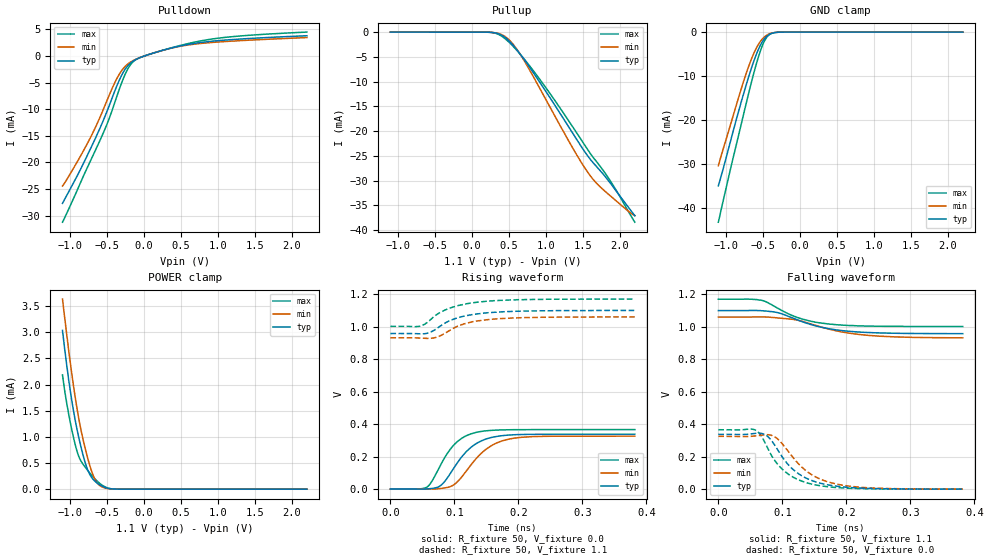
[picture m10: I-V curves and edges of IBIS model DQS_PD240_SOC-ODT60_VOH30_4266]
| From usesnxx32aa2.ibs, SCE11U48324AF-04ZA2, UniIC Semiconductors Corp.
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| DQS_PD240_SOC-ODT60_VOH30_4266
| (240 Ohm Pulldown, 60 Ohm System ODT Setting, VOH=VDDQ/3.0, 3200-4266Mbps)
[Model]   DQS_PD240_SOC-ODT60_VOH30_4266
Model_type   I/O
Vinl = 123.333mV
Vinh = 243.333mV
Vmeas = 183.333mV
Vref = 0.0mV
Cref = 0.0pF
Rref = 60.000Ohm
|   typ   min   max
|C_comp   0.838pF   0.788pF   0.888pF
C_comp_pullup   0.4190pF   0.3940pF   0.4440pF
C_comp_pulldown   0.4190pF   0.3940pF   0.4440pF
| Note: C_comp changes when the ODT circuit is enabled.
[Model Spec]
| Input threshold voltage corners
Vinl   0.1233V   0.1167V   0.1350V
Vinh   0.2433V   0.2367V   0.2550V
| Measurement voltage corners
Vmeas   0.1833V   0.1767V   0.1950V
| Timing spec test load voltage corners
Vref   0.0000V   0.0000V   0.0000V
| Dynamic Overshoot Parameters from LPDDR4 Specification
D_overshoot_ampl_h   0.30   NA   NA
D_overshoot_ampl_l   0.30   NA   NA
D_overshoot_area_h   0.1n   NA   NA
D_overshoot_area_l   0.1n   NA   NA
[Receiver Thresholds]
Vcross_low   = 123.3mV
Vcross_high  = 243.3mV
Vdiff_ac   = 120mV
Vdiff_dc   = 120mV
Tdiffslew_ac = 10.000ns |Not specified, so set to high value
[Voltage Range]   1.1000V   1.0600V   1.1700V
[Pullup Reference]   1.1000V   1.0600V   1.1700V
| Junction Temperature (Ambient temp is 35C typ 95C min -40C max)
[Temperature Range]   50.0   110.0   -40.0
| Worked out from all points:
|   slope of the pulldown table from 0 to 0.165 V, typ, clamps not added: 223 ohm
|   slope of the pullup table from 0 to 0.165 V, typ, clamps not added: 19.4 kohm
|   GND clamp passes 1 mA (typ) near -0.45 V on its own axis
|   POWER clamp passes 1 mA (typ) near -0.88 V on its own axis
|   rising waveform, R_fixture 50, V_fixture 0.0: 20-80 % time 41.5ps typ, 45.6ps min, 36.3ps max; typ from 0.001 V to 0.338 V
|   falling waveform, R_fixture 50, V_fixture 1.1: 20-80 % time 70.4ps typ, 79.9ps min, 60.1ps max; typ from 1.1 V to 0.958 V
|   rising waveform, R_fixture 50, V_fixture 1.1: 20-80 % time 51.9ps typ, 50ps min, 52.9ps max; typ from 0.958 V to 1.1 V
|   falling waveform, R_fixture 50, V_fixture 0.0: 20-80 % time 49.1ps typ, 53.6ps min, 45.1ps max; typ from 0.338 V to 0.001 V
[Pulldown]
|   Voltage   I(typ)   I(min)   I(max)
-1.1V     -27.71mA   -24.44mA   -31.25mA
-918.5mV  -22.98mA   -20.31mA   -25.78mA
-720.5mV  -17.39mA   -15.27mA   -19.65mA
-499.4mV  -10.41mA   -8.375mA   -12.82mA
-347.6mV  -5.002mA   -3.762mA   -6.827mA
-232.1mV  -2.055mA   -1.662mA   -2.791mA
-129.8mV  -798.7uA   -738.7uA   -879.6uA
0V        -19.07uA   -16.89uA   -13.69uA
394.9mV   1.594mA    1.561mA    1.646mA
843.7mV   2.68mA     2.468mA    3.039mA
1.395V    3.278mA    2.967mA    3.877mA
2.2V      3.818mA    3.475mA    4.505mA
[GND Clamp]
|   Voltage   I(typ)   I(min)   I(max)
-1.1V     -34.88mA   -30.34mA   -43.13mA
-944.9mV  -25.34mA   -21.53mA   -31.71mA
-789.8mV  -15.79mA   -12.83mA   -20.82mA
-723.8mV  -11.98mA   -9.381mA   -16.18mA
-664.4mV  -8.768mA   -6.598mA   -12.12mA
-588.5mV  -5.128mA   -3.689mA   -7.33mA
-522.5mV  -2.67mA    -1.906mA   -3.822mA
-466.4mV  -1.297mA   -942.8uA   -1.695mA
-413.6mV  -567.5uA   -419uA     -621.4uA
-354.2mV  -179.7uA   -135.9uA   -159.4uA
-258.5mV  -16.1uA    -14.2uA    -9.795uA
2.2V      0A         0A         0A
[Pullup]
|   Voltage   I(typ)   I(min)   I(max)
-1.1V     4.189uA    6.456uA    1.888uA
229.9mV   -30.52uA   -30.79uA   -31.1uA
332.2mV   -215.1uA   -179.7uA   -295.5uA
437.8mV   -961.7uA   -787.6uA   -1.21mA
553.3mV   -2.603mA   -2.4mA     -2.822mA
691.9mV   -5.249mA   -5.417mA   -5.187mA
1.075V    -13.73mA   -15.72mA   -12.85mA
1.411V    -21.61mA   -24.71mA   -20.28mA
1.576V    -25.28mA   -28.59mA   -24.04mA
1.695V    -27.39mA   -30.74mA   -26.42mA
1.89V     -30.93mA   -33.36mA   -30.56mA
2.2V      -37.14mA   -37.08mA   -38.43mA
[POWER Clamp]
|   Voltage   I(typ)   I(min)   I(max)
-1.1V     3.036mA    3.636mA    2.186mA
-1.041V   2.347mA    2.931mA    1.626mA
-981.2mV  1.754mA    2.277mA    1.183mA
-918.5mV  1.248mA    1.669mA    798.4uA
-859.1mV  857.6uA    1.195mA    561uA
-793.1mV  506.3uA    776.1uA    421uA
-740.3mV  306.1uA    494.5uA    324.3uA
-667.7mV  159.9uA    206.2uA    205.2uA
-598.4mV  83.67uA    71.98uA    113.1uA
-502.7mV  22.64uA    13.95uA    29.28uA
-400.4mV  2.596uA    1.715uA    2.318uA
2.2V      0A         0A         0A
[Ramp]
|   typ   min   max
| 20% - 80%
dV/dt_r   202.41m/41.49p   195.19m/45.58p   219.54m/36.31p
dV/dt_f   85.18m/70.36p   76.66m/80.11p   100.84m/60.22p
| 25% - 75%
|dV/dt_r   168.67m/33.07p   162.66m/36.29p   182.95m/28.91p
|dV/dt_f   70.98m/56.00p   63.88m/63.45p   84.03m/47.85p
R_load = 50
[Rising Waveform]
R_fixture = 50
V_fixture = 0.0
|   Time   V(typ)   V(min)   V(max)
0s        761.8uV    676.3uV    549.4uV
55ps      483uV      -90.77uV   8.246mV
63ps      3.123mV    -306.7uV   37.29mV
76ps      15.51mV    2.662mV    130.1mV
86ps      52.73mV    7.882mV    201.7mV
101ps     141mV      32.2mV     279.2mV
131ps     272.3mV    174.1mV    346.3mV
159ps     319mV      270.1mV    362mV
193ps     334.6mV    313.3mV    365.8mV
382ps     338.1mV    326mV      366.5mV
[Falling Waveform]
R_fixture   = 50
V_fixture   = 1.1
V_fixture_min = 1.06
V_fixture_max = 1.17
|   Time   V(typ)   V(min)   V(max)
0s        1.1V       1.06V      1.17V
47ps      1.1V       1.06V      1.171V
67ps      1.099V     1.061V     1.164V
90ps      1.09V      1.056V     1.121V
123ps     1.044V     1.041V     1.058V
146ps     1.013V     1.016V     1.033V
175ps     986.8mV    983.7mV    1.016V
206ps     971.8mV    960.1mV    1.008V
250ps     962.7mV    942.9mV    1.004V
382ps     958mV      932.2mV    1.002V
[Rising Waveform]
R_fixture   = 50
V_fixture   = 1.1
V_fixture_min = 1.06
V_fixture_max = 1.17
|   Time   V(typ)   V(min)   V(max)
0s        957.9mV    931.6mV    1.002V
45ps      955.8mV    930.2mV    1.002V
54ps      956.9mV    928.2mV    1.016V
68ps      977.1mV    930.9mV    1.061V
86ps      1.024V     961.1mV    1.104V
99ps      1.047V     991.2mV    1.122V
114ps     1.064V     1.016V     1.137V
140ps     1.081V     1.038V     1.153V
209ps     1.096V     1.056V     1.167V
382ps     1.1V       1.06V      1.17V
[Falling Waveform]
R_fixture = 50
V_fixture = 0.0
|   Time   V(typ)   V(min)   V(max)
0s        338.2mV    326.1mV    366.5mV
58ps      344.5mV    328.7mV    364mV
73ps      336.3mV    336.1mV    286.2mV
85ps      289.8mV    329.3mV    195.7mV
96ps      222.6mV    297.4mV    139.2mV
114ps     132.1mV    209mV      81.2mV
146ps     53.84mV    89.63mV    31.68mV
176ps     23.85mV    40.22mV    13.36mV
215ps     8.626mV    14.78mV    4.594mV
382ps     932.2uV    969uV      617uV
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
